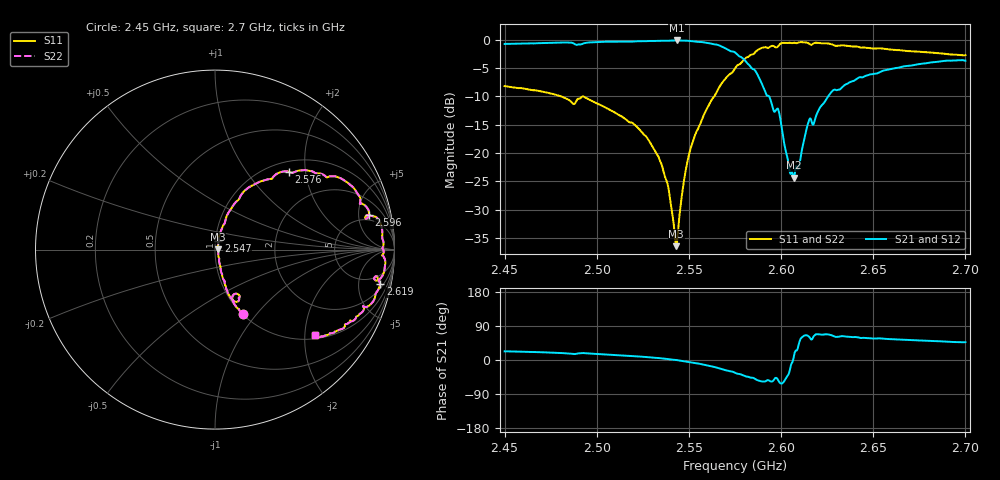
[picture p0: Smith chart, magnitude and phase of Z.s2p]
# Hz S dB R 50.0
!Frequency(Hz) S11_Amplitude(dB) S11_Phase(deg) S12_Amplitude(dB) S12_Phase(deg) S21_Amplitude(dB) S21_Phase(deg) S22_Amplitude(dB) S22_Phase(deg)
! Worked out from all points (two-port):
!   6311 points, 2.45 GHz to 2.7 GHz, reference 50 ohm
!   highest |S21| = -0.13 dB at 2.543 GHz (marker M1); lowest = -24.4 dB at 2.607 GHz (marker M2)
!   |S21| within 3 dB of the highest: start of sweep to 2.579 GHz
!   lowest |S11| = -36.5 dB at 2.543 GHz (marker M3), VSWR 1.03, Z = 51.5 + j0.0589 ohm
!   |S11| at or under -10 dB: 2.481 GHz to 2.564 GHz (83.2 MHz wide, 3.3 % of centre)
!   |S22| runs from -36.5 to -0.4 dB; largest |S21 - S12| = 5.1e-06
!   S11 on the Smith chart (normalised r, x): 2.45 GHz: 1.01, -0.85; 2.547 GHz: 1.03, +0.10; 2.576 GHz: 1.20, +1.62; 2.596 GHz: 4.01, +6.78; 2.619 GHz: 2.61, -8.85; 2.7 GHz: 1.09, -2.24
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2.45e9  -8.19 -66.6  -0.74 22.9  -0.74 22.9  -8.19 -66.6
2.491665e9  -10.11 -64.6  -0.81 18.0  -0.81 18.0  -10.11 -64.6
2.520037e9  -14.87 -73.7  -0.31 10.3  -0.31 10.3  -14.87 -73.7
2.533424e9  -20.63 -72.4  -0.21 5.2  -0.21 5.2  -20.63 -72.4
2.538831e9  -26.12 -64.7  -0.18 2.6  -0.18 2.6  -26.12 -64.7
2.543111e9  -36.46 2.2  -0.13 -0.0  -0.13 -0.0  -36.46 2.2
2.5434e9  -36.15 16.2  -0.13 -0.3  -0.13 -0.3  -36.15 16.2
2.546808e9  -26.01 68.8  -0.15 -2.7  -0.15 -2.7  -26.01 68.8
2.550161e9  -20.13 73.0  -0.21 -5.5  -0.21 -5.5  -20.13 73.0
2.556366e9  -14.67 70.6  -0.40 -10.5  -0.40 -10.5  -14.67 70.6
2.575001e9  -5.06 50.2  -2.25 -33.7  -2.25 -33.7  -5.06 50.2
2.576476e9  -4.46 46.6  -2.71 -36.4  -2.71 -36.4  -4.46 46.6
2.58814e9  -1.66 27.0  -6.78 -54.9  -6.78 -54.9  -1.66 27.0
2.595919e9  -1.11 12.5  -12.50 -53.5  -12.50 -53.5  -1.11 12.5
2.601334e9  -0.56 6.8  -17.67 -58.3  -17.67 -58.3  -0.56 6.8
2.604569e9  -0.54 2.1  -23.14 -29.9  -23.14 -29.9  -0.54 2.1
2.60684e9  -0.54 -0.4  -24.37 6.9  -24.37 6.9  -0.54 -0.4
2.616718e9  -0.87 -9.6  -14.64 54.3  -14.64 54.3  -0.87 -9.6
2.618843e9  -0.53 -11.9  -13.59 67.8  -13.59 67.8  -0.53 -11.9
2.627115e9  -0.78 -20.0  -9.31 65.7  -9.31 65.7  -0.78 -20.0
2.658371e9  -1.70 -33.1  -5.26 55.3  -5.26 55.3  -1.70 -33.1
2.699988e9  -2.70 -40.7  -3.70 47.0  -3.70 47.0  -2.70 -40.7
